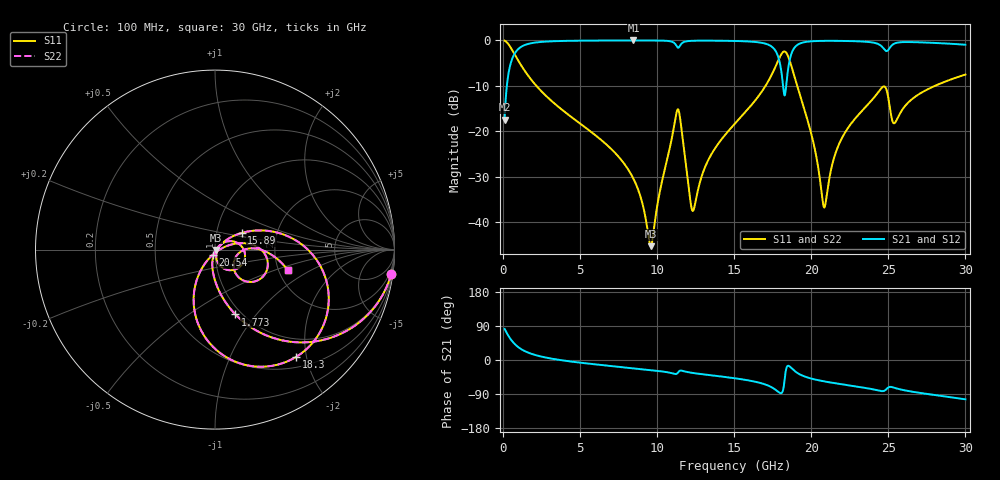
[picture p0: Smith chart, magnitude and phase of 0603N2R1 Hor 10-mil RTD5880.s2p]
# GHz S MA R 50
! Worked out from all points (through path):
!   3201 points, 100 MHz to 30 GHz, reference 50 ohm
!   highest |S21| = -0.04 dB at 8.463 GHz (marker M1); lowest = -17.5 dB at 100 MHz (marker M2)
!   group delay of S21, straight-line fit = 11 ps
!   lowest |S11| = -45.3 dB at 9.584 GHz (marker M3), VSWR 1.01, Z = 50.5 - j0.28 ohm
!   |S11| at or under -10 dB: 2.153 GHz to 17.04 GHz (14.88 GHz wide, 155 % of centre); 19.08 GHz to 28.04 GHz (8.961 GHz wide, 38 % of centre)
!   |S22| runs from -45.3 to -0.1 dB; largest |S21 - S12| = 0
!   S11 on the Smith chart (normalised r, x): 100 MHz: 1, -14; 1.773 GHz: 0.94, -0.79; 15.89 GHz: 1.32, +0.25; 18.3 GHz: 0.67, -1.82; 20.54 GHz: 0.97, -0.06; 30 GHz: 2.24, -0.61
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0.1  0.991 -8.0  0.1339 82.0  0.1339 82.0  0.991 -8.0
0.6139062  0.7687 -41.4  0.639 48.5  0.639 48.5  0.7687 -41.4
1.772531  0.3785 -72.5  0.9241 17.3  0.9241 17.3  0.3785 -72.5
5.089563  0.118 -96.1  0.9903 -7.4  0.9903 -7.4  0.118 -96.1
8.462656  0.02986 -104.0  0.9953 -21.8  0.9953 -21.8  0.02986 -104.0
9.583906  0.005422 -30.8  0.9945 -26.6  0.9945 -26.6  0.005422 -30.8
10.06978  0.01755 37.7  0.9927 -28.9  0.9927 -28.9  0.01755 37.7
11.3125  0.1718 -13.2  0.8383 -35.0  0.8383 -35.0  0.1718 -13.2
12.32162  0.01324 -18.5  0.9871 -34.2  0.9871 -34.2  0.01324 -18.5
15.05  0.1213 37.0  0.9824 -48.3  0.9824 -48.3  0.1213 37.0
15.89094  0.1747 32.0  0.971 -53.6  0.971 -53.6  0.1747 32.0
17.55412  0.4608 5.8  0.8161 -75.0  0.8161 -75.0  0.4608 5.8
18.30163  0.7494 -52.9  0.2544 -41.0  0.2544 -41.0  0.7494 -52.9
18.86225  0.4248 -102.8  0.8066 -27.0  0.8066 -27.0  0.4248 -102.8
20.03956  0.08775 -125.7  0.9752 -49.4  0.9752 -49.4  0.08775 -125.7
20.54413  0.03096 -113.1  0.9834 -54.1  0.9834 -54.1  0.03096 -113.1
20.87116  0.01466 -43.8  0.9854 -56.6  0.9854 -56.6  0.01466 -43.8
22.24469  0.09994 17.1  0.9822 -65.6  0.9822 -65.6  0.09994 17.1
24.60866  0.304 -14.5  0.8439 -82.2  0.8439 -82.2  0.304 -14.5
25.01978  0.2217 -48.5  0.7924 -71.9  0.7924 -71.9  0.2217 -48.5
25.41222  0.1228 -19.5  0.9226 -73.5  0.9226 -73.5  0.1228 -19.5
30  0.4195 -15.6  0.8939 -103.7  0.8939 -103.7  0.4195 -15.6
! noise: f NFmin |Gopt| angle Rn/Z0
0.1  0.0004461  0.948  0.9117  0.001923
3.417  0.004026  0.8096  9.819  0.004373
6.743  0.006939  0.7858  18.92  0.006483
10.06  0.0123  0.8178  27.9  0.01331
13.39  0.01554  0.8107  36.84  0.01542
16.7  0.02918  0.8715  45.54  0.04162
20.03  0.02992  0.853  54.38  0.0344
23.35  0.0287  0.8262  62.53  0.02546
26.67  0.03214  0.8251  70.67  0.02582
30  0.03022  0.797  78.25  0.01869
